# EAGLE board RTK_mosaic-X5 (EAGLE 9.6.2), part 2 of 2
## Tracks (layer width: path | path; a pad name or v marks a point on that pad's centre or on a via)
1.8V  (via drill 0.3)
  Top 0.254: C60.1 51.88,78.02 51.88,86.61 52.69,87.42 U13.1 | R18.2 92.9,89.11 | 92.9,89.11 93.88,89.11 94.41,89.65 U11.5 | U11.1 92.91,89.1 92.9,89.11
  Top 0.406: v63.18,74.42 57.25,74.42 C62.1 C60.1
  Top 0.61: U8.AC4 89.85,86.36 1V8.1 90.07,89.11 R18.2
  Route15 0.61: 1V8.1 84.77,87.63 71.56,74.42 v63.18,74.42
2V8
  Top 0.152: U8.M23 U8.N23 63.18,71.12 2V8.1
3.3V  (via drill 0.3)
  Top 0.152: U7.17 135.09,62.87 v135.06,62.84
  Top 0.254: R16.2 127.74,52.2 v127.44,52.2 | R59.1 v8.57,16.51 | R58.1 v132.78,70.23 | R57.1 v131.25,75.69 | U17.1 100.53,88.89 v100.52,88.9 | U17.5 102.03,88.91 v102.04,88.9 | U18.1 104.34,88.89 v104.33,88.9 | U4.P2 v111.19,88.9
  Top 0.406: C1.1 109.74,78.32 R3.2 | v122.24,28.07 122.24,27.09 C3.1 C4.1 122.28,24.42 v122.24,24.38 U2.16 | U2.4 v126.05,18.8 | U6.1 73.22,39.03 73.3,38.95
  Top 0.61: J4.2 76.38,13.2 v76.71,13.53 77.15,13.97 80.84,13.97 81.34,14.48 C56.1
  Top 0.813: 3V3.1 77.57,38.95 C15.1 C14.1 73.3,38.95 | v141.29,57.15 C32.1 | C32.1 C21.1 FB2.1 | R21.2 v131.89,57.15 131.09,57.15 R49.2 | 112.42,76.62 C1.1 111.44,67.31 110.35,66.22 U1.2 | 112.42,76.62 v112.46,76.58 | 112.42,76.62 C2.1 114.45,76.62 v114.49,76.58 | VCCIO.1 117.79,86.69 117.79,88.01 | 117.79,88.01 v117.79,88.9 v119.06,88.9 | v82.61,28.07 v82.61,26.67 82.61,16.04 82.23,15.66 C56.1 | C32.1 R29.2 | C41.1 117.75,88.05 117.79,88.01
  Route15 0.152: v135.06,62.84 135.06,57.15
  Route15 0.254: v8.57,16.51 10.35,18.29 26.86,18.29 40.83,4.32 53.53,4.32 62.74,13.53 v76.71,13.53 | v132.78,70.23 131.89,70.23 | v131.25,75.69 129.67,74.11
  Route15 0.813: v126.05,18.8 126.05,19.68 122.24,23.5 v122.24,24.38 v122.24,28.07 122.24,38.1 | 3V3.1 82.61,38.1 | 82.61,38.1 122.24,38.1 | 122.24,38.1 129.22,38.1 131.89,40.77 131.89,52.2 | v141.29,57.15 135.06,57.15 v131.89,57.15 | v112.46,76.58 v114.49,76.58 127.19,76.58 | 131.89,52.2 v131.89,57.15 | v127.44,52.2 131.89,52.2 | 125.41,88.9 127.19,87.12 127.19,76.58 | 125.41,88.9 v119.06,88.9 v117.79,88.9 v111.19,88.9 v104.33,88.9 v102.04,88.9 v100.52,88.9 | 125.41,88.9 125.41,97.79 126.68,99.06 132.78,99.06 | 132.78,99.06 140.67,99.06 J9.11 | J9.13 132.75,99.03 132.78,99.06 | 127.19,76.58 129.67,74.11 131.89,71.88 131.89,70.23 v131.89,57.15 | v82.61,26.67 v82.61,28.07 82.61,38.1
  Bottom 0.152: I2C.2 75.88,14.35 v76.71,13.53
  Bottom 0.813: ESP2.1 104.2,76.58 v112.46,76.58 v114.49,76.58
  cutout Route15: 22.8,91.06 arc-90 24.7,89.15 arc-90 22.8,87.25 arc-90 20.89,89.15 arc-90
3.3V_SW  (via drill 0.3)
  Top 0.152: U8.B8 84.14,57.78 72.07,57.78 | R56.1 34.23,87.03 v34.23,88.27 | R55.1 R15.2 | U14.1 45.92,88.15 47.42,89.65 U14.5
  Top 0.254: v45.91,77.09 45.81,76.99 U9.17 | U16.1 96.72,88.89 v96.71,88.9 | v44.01,87.25 44.89,87.25 45.07,87.42 U14.1 | U15.1 48.88,87.42 v48.7,87.25
  Top 0.406: J3.4 45.62,13.88 44.77,14.73 44.77,15.62 C18.1 44.75,15.68 D34.1 42.16,15.68 v42.1,15.62 42.1,17.02 41.76,17.36 R47.2 | U3.1 73.05,44.11 73.13,44.03 | U8.C18 v72.07,69.85 | C63.1 98.02,83.22 v97.35,82.55 97.35,76.33 RDY1.1 | R46.2 v52.13,18.41 55.18,18.41 55.44,18.16 R17.2
  Top 0.61: C54.1 68.77,53.34 69.53,54.1 U8.A20 U8.B20 U8.C20 | C53.1 70.42,53.34 70.8,53.72 U8.A19 U8.B19 U8.C19 | C46.1 U8.A18 U8.B18 72.07,57.78 U8.C18
  Top 0.813: C7.1 C6.1 73.13,44.03 | C7.1 77.57,44.03 3V3_SW.1 | C7.1 76.39,50.29 75.03,51.65 C46.1 C53.1 C54.1 | v49.34,15.62 48.11,15.62 C19.1 C20.1 C18.1 | FB1.1 48.83,70.32 v48.83,68.58 | v37.02,67.31 R20.2 | C5.1 v45.91,77.09 | C11.1 v45.91,78.74 | R15.2 v44.01,87.25 | C58.1 v42.35,87.25
  Route15 0.813: 3V3_SW.1 78.42,40.64 77.53,39.75 60.26,39.75 | v42.1,15.62 v49.34,15.62 v52.13,18.41 60.26,26.54 60.26,39.75 | 60.26,39.75 58.1,41.91 58.1,51.31 48.83,60.58 v48.83,68.58 45.91,68.58 | 45.91,68.58 38.29,68.58 v37.02,67.31 | 45.91,68.58 v45.91,77.09 v45.91,78.74 45.91,87.25 | 45.91,87.25 v44.01,87.25 v42.35,87.25 34.73,87.25 34.23,87.76 v34.23,88.27 34.23,89.28 32.07,91.44 26.37,91.44 J2.11 18.75,99.06 13.63,99.06 J2.13 | 45.91,87.25 v48.7,87.25
  Bottom 0.406: v72.07,69.85 74.61,69.85 87.31,82.55 v97.35,82.55 97.35,83.44 96.71,84.07 v96.71,88.9
5V  (via drill 0.3)
  Top 0.152: U6.5 67.84,40.98 67.09,40.23 67.09,39.05 | U3.5 67.97,46.06 67.09,45.19 67.09,44.13
  Top 0.406: U3.8 67.9,44.11 | U6.8 67.9,39.03 67.88,39.05
  Top 0.61: U8.A8 v84.77,53.34
  Top 0.813: 67.88,39.05 67.09,39.05 C17.1 62.33,38.95 60.64,40.64 5V.1 | 67.09,44.13 C9.1 | C9.1 C8.1 C10.1 61.06,44.03 5V.1 | F1.1 54.78,47.78 56.69,45.86 C57.+ 5V.1 | v56.83,73.41 v58.1,73.41 FB3.1 | v84.77,53.34 v83.63,53.34 82.87,53.34 82.23,52.7 C61.1 | v125.41,86.61 v124.14,86.61 122.86,86.61 VCCIO.3 | C9.1 67.07,44.11 67.9,44.11
  Route15 0.813: 5V.1 60.64,53.34 | 60.64,53.34 58.1,55.88 v58.1,73.41 v56.83,73.41 | 60.64,53.34 v83.63,53.34 v84.77,53.34 103.31,53.34 104.46,54.48 104.46,81.92 105.09,82.55 122.87,82.55 125.41,85.09 v125.41,86.61 v124.14,86.61
5V_RAW
  Top 0.813: U10.2 U10.1 29.72,54.17 30.3,54.75 C48.+ 32.93,54.98 C49.1 | C49.1 C50.1 | L1.1 37.78,53.38 C49.1
5V_RAW1
  Top 0.813: C16.+ 41.96,26.9 C51.1 C84.1 42.06,33.76 L4.1
  Top 1.905: U12.4 C16.+
!BOOT!  (via drill 0.3)
  Top 0.152: R16.1 R19.2 v134.3,51.18 | Q1.6 115.9,18.91 116.01,18.8 116.4,18.8 v116.52,18.92 | v121.6,20.32 v139.38,20.32
  Bottom 0.152: BOOT_SW.1 TP_BOOT.1 v139.38,20.32 139.38,46.1 v134.3,51.18 | v116.52,18.92 120.2,18.92 v121.6,20.32
!RESET!  (via drill 0.3)
  Top 0.152: MOSAIC_RST.4 v97.47,43.18 102.55,38.1 v102.55,21.59 | U1.3 106.29,64.95 v106.24,64.9 106.24,75.22 C31.1 R3.1 | Q1.3 114.6,21.86 114.36,22.1 113.22,22.1 v112.71,21.59
  Bottom 0.152: v97.47,43.18 100.01,45.72 100.01,64.01 100.9,64.9 v106.24,64.9 | RESET_SW.1 112.71,13.22 v112.71,21.59 v102.55,21.59 | MOSAIC_RST.4 MOSAIC_RST.2
ANT1
  Top 0.318: ANT1.SIG 69.53,94.69 D17.1 arc90 69.49,94.5 L3.2 69.49,83.86 arc90 U8.AC20
ANT2
  Top 0.318: U8.V23 64.92,77.47 arc-90 62.38,80.01 R53.2 62.37,81.3 D2.1 62.33,85.38 L2.1 62.42,87.08 ANT2.FEED
CH340-DTR  (via drill 0.3)
  Top 0.152: R4.2 117.72,21.24 v116.78,21.24 Q1.1 115.9,22.21 115.25,22.86 DTR.1 | U2.13 126.05,21.84 125.41,21.21 v120.33,21.21
  Bottom 0.152: v120.33,21.21 116.81,21.21
  Bottom 0.267: 116.81,21.21 v116.78,21.24
CH340-RTS  (via drill 0.3)
  Top 0.152: R5.2 111.51,19.4 v113.47,19.4 Q1.4 114.6,18.43 115.25,17.78 RTS.1 | U2.14 124.78,22.23 124.4,21.85 119.96,21.85 119.19,21.08 v119.19,19.43
  Bottom 0.152: 119.16,19.4 v113.47,19.4
  Bottom 0.267: v119.19,19.43 119.16,19.4
CH340-RXI  (via drill 0.3)
  Top 0.152: U2.3 124.78,15.88 TX.1 | v120.97,49.66 120.21,49.66 119.7,50.16 119.7,60.33 123.05,63.68 U1.35
  Bottom 0.152: v120.97,49.66 120.97,44.58 127.19,38.35 127.19,17.27 125.41,15.49 TX.1
CH340-TXO  (via drill 0.3)
  Top 0.152: U2.2 123.51,15.88 RX.1 | v120.33,50.8 120.33,60.33 122.42,62.41 U1.34
  Bottom 0.152: v120.33,50.8 120.33,44.45 126.68,38.1 126.68,18.03 123.89,15.24 RX.1
COM2_CTS
  Top 0.152: U8.J1 COM2_CTS.1
COM2_RTS
  Top 0.152: U8.G1 COM2_RTS.1
COM2_RX
  Top 0.152: U8.F1 COM2_RX.1
COM2_TX
  Top 0.152: U8.H1 COM2_TX.1
COM3_CTS
  Top 0.152: U8.N1 97.47,71.12 COM3_CTS.1
COM3_RTS
  Top 0.152: U8.L1 97.47,68.58 COM3_RTS.1
COM3_RX
  Top 0.152: U8.K1 COM3_RX.1
COM3_TX
  Top 0.152: U8.M1 96.96,69.85 98.23,71.12 COM3_TX.1
COM4_RX  (via drill 0.3)
  Top 0.152: U8.D3 91.76,59.05 96.58,59.05 100.52,55.12 v101.79,55.12 | v133.03,47.88 R52.2
  Bottom 0.152: v101.79,55.12 133.41,55.12 133.67,54.86 133.67,48.51 v133.03,47.88
COM4_TX  (via drill 0.3)
  Top 0.152: U8.E3 91.76,60.33 96.2,60.33 100.65,55.88 v101.79,55.88 | v132.91,55.63 132.1,55.63 130.96,54.48 R51.2
  Bottom 0.152: v101.79,55.88 131.64,55.88 131.89,55.63 v132.91,55.63
D+_ESP32  (via drill 0.3)
  Top 0.152: 127.7,8.89 J1.A6 127.7,5.33 127.95,5.08 128.46,5.08 128.7,5.32 J1.B6
  Top 0.267: 127.7,8.89 127,9.59 D10.1 127,11.37 v127.19,11.56 | v127.44,16.51 127.44,16.63 127.32,16.76 U2.5
  Bottom 0.267: v127.44,16.51 127.7,16.26 127.7,12.06 v127.19,11.56
D+_MOSAIC
  Top 0.267: J6.A6 104.84,5.2 104.97,5.08 105.6,5.08 105.84,5.32 J6.B6 105.84,7.8 107.25,9.21 107.25,11.05 106.04,12.26 D8.1 106.04,13.78 105.38,14.45 105.38,14.95 105.49,15.07 T1.A2
D+_MOSAIC_T
  Top 0.267: U8.A5 88.58,55.63 105.35,38.86 105.35,18.16 105.49,18.02 T1.A1
D-_ESP32  (via drill 0.3)
  Top 0.152: J1.B7 127.19,6 v127.19,7.11 | 128.2,8.89 128.2,7.24 v128.33,7.11 128.2,6.98 J1.A7
  Top 0.267: 128.2,8.89 128.9,9.59 D10.3 128.9,11.37 v128.71,11.56 | v128.46,16.51 128.59,16.64 U2.6
  Bottom 0.152: v128.33,7.11 v127.19,7.11
  Bottom 0.267: v128.46,16.51 128.21,16.26 128.21,12.06 v128.71,11.56
D-_MOSAIC
  Top 0.267: J6.A7 105.34,6.99 | 105.34,6.99 105.34,8 106.73,9.38 106.73,10.82 105.87,11.68 104.33,11.68 104.14,11.87 D8.3 104.14,13.78 104.81,14.45 104.81,14.95 104.69,15.07 T1.B2 | J6.B7 104.34,6.74 104.58,6.99 105.34,6.99
D-_MOSAIC_T
  Top 0.267: T1.B1 104.69,17.95 104.84,18.1 104.84,38.61 87.57,55.88 U8.A6
ESP2_TX
  Top 0.152: U1.24 125.7,49.53 R48.1 R52.1
ESP4_RX
  Top 0.152: U1.26 126.48,52.25 127.06,52.83 127.06,54.23 127.32,54.48 R51.1
ESP5_ERST  (via drill 0.3)
  Top 0.152: U1.29 128.3,56.06 R49.1 128.37,57.19 129.6,58.42 v130.49,58.42 | U7.32 139.74,67.79 139.89,67.94 v140.65,67.94
  Bottom 0.152: v130.49,58.42 133.03,60.96 139.38,60.96 141.16,62.74 141.16,67.44 v140.65,67.94
ESP12_LED_WIFI  (via drill 0.3)
  Top 0.152: v104.58,49.4 104.58,50.71 R50.1 104.85,50.98 U1.14 | v10.22,15.98 R28.1
  Bottom 0.152: v104.58,49.4 104.58,47.62 97.6,40.64 85.79,40.64 58.48,13.34 16.68,13.34 14.03,15.98 v10.22,15.98
ESP14_SCL  (via drill 0.3)
  Top 0.152: R_SCL.1 71.35,16.38 v70.8,16.38 | J4.4 73.2,11.93 72.71,11.43 SCL2.1 | v106.11,52.32 107.45,52.32 U1.13 | v73.98,16.38 73.98,26.04 89.85,41.91 v96.96,41.91 | v100.77,45.72 100.77,51.56 101.54,52.32 v103.95,52.32 104.3,52.68 104.3,77.64 106.95,80.29 107.52,80.29 111.69,84.47 U4.P3
  Bottom 0.152: v73.98,16.38 v70.8,16.38 SCL2.1 | v103.95,52.32 v106.11,52.32 | v100.77,45.72 v96.96,41.91
ESP14_SCL_IO  (via drill 0.3)
  Top 0.152: R_SCL_IO.1 110.3,85.98 v110.68,85.6 | U4.P6 111.69,92.27 D26.1
  Top 0.406: J13.4 112.88,94.53 111.75,93.4 D26.1
  Bottom 0.152: v110.68,85.6 112.88,87.8 J13.4
ESP15_LED_BT  (via drill 0.3)
  Top 0.152: v105.22,48.51 107.45,48.51 U1.16 | R36.1 13.23,14.82 v13.65,15.24
  Bottom 0.152: v13.65,15.24 15.94,12.95 58.61,12.95 85.92,40.26 97.98,40.26 105.22,47.5 v105.22,48.51
ESP15_SDA  (via drill 0.3)
  Top 0.152: 78.42,15.66 78,15.66 74.36,19.3 74.36,26.02 89.74,41.4 v97.6,41.4 | 78.42,15.66 R_SDA.1 | J4.3 75.38,11.04 75.59,10.83 80.36,10.83 SDA2.1 | v78.42,15.7 78.42,15.66 | v124.14,48.39 125.47,48.39 U1.23 | v101.28,45.09 101.28,51.56 101.54,51.82 104.33,51.82 105.09,52.58 v105.09,52.96 104.58,53.47 104.58,77.52 107.07,80.01 107.63,80.01 112.19,84.57 U4.P4
  Bottom 0.152: SDA2.1 78.42,13.97 v78.42,15.7 | v105.09,52.96 119.57,52.96 v124.14,48.39 | v101.28,45.09 v97.6,41.4
ESP15_SDA_IO  (via drill 0.3)
  Top 0.152: R_SDA_IO.1 110.3,84.33 v110.68,84.71 | U4.P5 112.19,91.05 112.59,91.44 113.47,91.44 114.36,92.33 D25.1
  Top 0.406: D25.1 115.18,93.27 116.38,94.47 J13.3
  Bottom 0.152: v110.68,84.71 116.38,90.41 J13.3
ESP18_MDIO  (via drill 0.3)
  Top 0.152: U7.11 133.3,66.79 v133.29,66.8 | v130.87,63.5 131.34,63.5 131.89,62.95 R21.1 131.09,60.54 127.88,57.33 U1.30
  Bottom 0.152: v133.29,66.8 130.87,64.39 v130.87,63.5
ESP19_TXD0  (via drill 0.3)
  Top 0.152: U1.31 126.61,58.6 126.81,58.8 126.81,60.07 128.71,61.98 v130.24,61.98 | U7.24 138.59,62.58 v138.37,62.36
  Bottom 0.152: v130.24,61.98 130.37,61.85 137.86,61.85 v138.37,62.36
ESP21_TXEN  (via drill 0.3)
  Top 0.152: U1.33 127.24,61.14 128.59,62.48 v130.87,62.48 | v137.73,62.74 138.09,63.1 U7.23
  Bottom 0.152: v137.73,62.74 137.22,62.23 131.13,62.23 v130.87,62.48
ESP22_TXD1  (via drill 0.3)
  Top 0.152: U1.36 126.63,64.95 128.59,62.99 v130.24,62.99 | v140.53,64.26 139.25,64.26 U7.25
  Bottom 0.152: v130.24,62.99 131.51,62.99 131.89,63.37 139.64,63.37 v140.53,64.26
ESP23_MDC
  Top 0.152: U1.37 126.5,66.22 128.59,64.14 131.89,64.14 132.52,64.77 132.52,65.41 133.41,66.29 U7.12
ESP25_RXD0  (via drill 0.3)
  Top 0.152: U1.10 108.96,56.06 v109.28,56.39 | v135.19,56.26 R30.1
  Bottom 0.152: v109.28,56.39 109.41,56.26 133.03,56.26 133.54,55.75 134.68,55.75 v135.19,56.26
ESP26_RXD1  (via drill 0.3)
  Top 0.152: U1.11 108.57,54.79 v110.81,57.02 | R31.1 133.54,56.72 v133.92,56.34
  Bottom 0.152: v110.81,57.02 111.16,56.67 133.03,56.67 133.36,56.34 v133.92,56.34
ESP27_CRSDV  (via drill 0.3)
  Top 0.152: U1.12 109.08,53.52 v110.17,54.61 | v132.91,54.61 133.92,55.63 135.57,55.63 136.08,56.13 136.08,57.06 136.84,57.82 R32.1
  Bottom 0.152: v110.17,54.61 v132.91,54.61
ESP32_RF
  Top 0.318: ESP32_RF.SIG 82.23,94.67 D3.1 82.18,92.44 J8.FEED
ESP32_TX  (via drill 0.3)
  Top 0.152: v102.55,59.31 103.34,60.1 103.34,81.76 101.03,84.07 U17.2 | v106.11,58.67 107.45,58.67 U1.8
  Bottom 0.152: v106.11,58.67 105.35,57.91 103.31,57.91 102.55,58.67 v102.55,59.31
ESP32_TX_O
  Top 0.152: U17.7 101.03,91.32 101.16,91.44 102.17,91.44 102.37,91.64 D24.1
  Top 0.406: D24.1 102.37,95.61 J13.7
ESP33_RTS  (via drill 0.3)
  Top 0.152: v102.55,57.4 102.55,58.55 103.62,59.61 103.62,81.99 101.53,84.08 U17.3 | v106.11,57.4 107.45,57.4 U1.9
  Bottom 0.152: v102.55,57.4 v106.11,57.4
ESP33_RTS_O
  Top 0.152: U17.6 101.53,90.93 101.66,91.06 103.5,91.06 D23.1
  Top 0.406: D23.1 104.77,93.27 105.88,94.39 J13.6
ESP34_RX  (via drill 0.3)
  Top 0.152: v102.55,61.85 103.06,62.36 103.06,81.28 v102.43,81.92 | v106.11,61.09 107.47,61.09 U1.6 | U18.2 v104.84,84.33
  Bottom 0.152: v102.55,61.85 105.35,61.85 v106.11,61.09 | v102.43,81.92 v104.84,84.33
ESP34_RX_I  (via drill 0.3)
  Top 0.152: U18.7 104.84,91.11 v104.87,91.14
  Top 0.406: D28.1 98.81,95.56 J13.8
  Bottom 0.152: v104.87,91.14 99.93,91.14 98.88,92.19 J13.8
ESP35_CTS  (via drill 0.3)
  Top 0.152: v103.44,58.67 103.95,59.18 103.95,82.68 105.34,84.07 U18.3 | v106.11,59.94 107.45,59.94 U1.7
  Bottom 0.152: v103.44,58.67 104.84,58.67 v106.11,59.94
ESP35_CTS_I
  Top 0.152: U18.6 105.34,90.8 105.73,91.19 106.36,91.19 107.51,92.33 D27.1
  Top 0.406: D27.1 108.32,93.4 109.38,94.46 J13.5
ESP36  (via drill 0.3)
  Top 0.152: v105.47,63.63 105.53,63.68 U1.4
  Bottom 0.152: ESP36.1 101.28,61.98 101.79,62.48 104.33,62.48 v105.47,63.63
ESP39  (via drill 0.3)
  Top 0.152: U1.5 105.91,62.41 105.35,61.85 v105.35,60.45
  Bottom 0.152: v105.35,60.45 102.68,60.45 102.04,59.82 101.54,59.82 101.28,59.56 ESP39.1
ESP_REFCLK  (via drill 0.3)
  Top 0.152: R19.1 128.17,50.98 U1.25 123.96,50.98 122.87,52.07 v122.87,59.69 | v133.41,67.77 134.45,67.77 U7.9
  Bottom 0.152: v122.87,59.69 127.95,59.69 129.6,61.34 129.6,63.96 v133.41,67.77
ETHER_!RST!  (via drill 0.3)
  Top 0.152: U9.32 39.84,81.66 v39.56,81.94 | v42.35,82.93 R22.2 | U8.F2 91.76,62.87 90.61,62.87 90.11,63.37 v88.58,63.37 | v53.02,63.37 53.02,68.2 49.53,71.69 v49.15,71.69
  Bottom 0.152: v39.56,81.94 41.34,81.94 42.33,82.93 v42.35,82.93 44.89,82.93 49.15,78.68 v49.15,71.69 | v88.58,63.37 v53.02,63.37
ETHER_CLK  (via drill 0.3)
  Top 0.152: U8.AA2 91.76,80.64 90.49,80.64 90.11,80.26 90.11,78.99 81.85,70.74 v81.85,67.56 | U9.9 39.84,74.65 40.2,74.3 43.24,74.3 44.64,75.69 50.61,75.69 56.45,69.85 v56.96,69.85
  Bottom 0.152: v81.85,67.56 81.47,67.18 57.59,67.18 57.34,67.44 57.34,69.47 v56.96,69.85
ETHER_CRSDV  (via drill 0.3)
  Top 0.152: v55.05,66.67 54.93,66.8 54.93,68.83 49.85,73.91 45.4,73.91 44.01,72.52 v44.01,72.26 | U8.N2 91.76,71.75 89.47,71.75 85.28,67.56 v85.28,65.66 | U9.18 44.66,77.49 v44.77,77.6
  Bottom 0.152: v85.28,65.66 85.28,65.53 85.03,65.28 55.69,65.28 55.44,65.53 55.44,66.29 v55.05,66.67 | v44.01,72.26 44.01,76.83 v44.77,77.6
ETHER_MDC  (via drill 0.3)
  Top 0.152: v83.38,66.8 83.38,70.36 89.85,76.83 91.76,76.83 U8.V2 | v41.59,73.28 43.24,73.28 45.02,75.06 50.24,75.06 56.07,69.23 56.07,68.71 v56.2,68.58 | U9.12 41.34,75.18 v41.59,74.93
  Bottom 0.152: v83.38,66.8 82.99,66.42 56.83,66.42 56.58,66.67 56.58,68.2 v56.2,68.58 | v41.59,74.93 | v41.59,73.28 v41.59,74.93
ETHER_MDIO  (via drill 0.3)
  Top 0.152: U8.W2 91.76,78.11 90.11,78.11 82.61,70.61 v82.61,67.18 | v56.58,69.24 50.48,75.34 44.77,75.34 43.24,73.81 v40.96,73.81 40.93,73.79 39.18,73.79 37.02,71.63 R20.1 | v40.83,75.56 40.83,76.35 U9.11
  Bottom 0.152: v56.58,69.24 56.96,68.86 56.96,67.08 57.21,66.83 82.33,66.83 82.61,67.11 v82.61,67.18 | v40.96,73.81 40.96,75.44 v40.83,75.56
ETHER_RXD0  (via drill 0.3)
  Top 0.152: U8.R2 91.76,73.03 89.85,73.03 84.65,67.82 v84.65,66.04 | v55.44,67.31 55.31,67.44 55.31,68.96 49.97,74.3 45.28,74.3 43.24,72.26 v42.74,72.26 | v43.5,75.44 43.34,75.59 U9.16
  Bottom 0.152: v84.65,66.04 84.26,65.66 62.29,65.66 56.07,65.66 55.82,65.91 55.82,66.93 v55.44,67.31 | v43.5,75.44 43.5,73.03 v42.74,72.26
ETHER_RXD1  (via drill 0.3)
  Top 0.152: U8.T2 91.76,74.3 90.23,74.3 84.01,68.07 v84.01,66.42 | v42.23,72.77 43.24,72.77 45.15,74.68 50.1,74.68 55.69,69.09 55.69,68.07 v55.82,67.94 | v42.86,74.93 42.84,74.95 U9.15
  Bottom 0.152: v84.01,66.42 84.01,66.35 83.73,66.07 56.42,66.07 56.2,66.29 56.2,67.56 v55.82,67.94 | v42.86,74.93 42.23,74.3 v42.23,72.77
ETHER_RXER  (via drill 0.3)
  Top 0.152: U8.M2 91.76,70.48 89.09,70.48 86.04,67.44 v86.04,65.28 | v44.89,72.26 44.89,72.9 45.53,73.53 49.72,73.53 54.55,68.71 54.55,66.17 v54.67,66.04 | U9.20 v44.76,78.49 v44.77,78.49
  Bottom 0.152: v86.04,65.28 85.66,64.9 55.31,64.9 55.05,65.15 55.05,65.66 v54.67,66.04 | v44.77,78.49 45.28,77.98 45.28,72.64 v44.89,72.26
ETHER_TXD0  (via drill 0.3)
  Top 0.152: U9.24 44.87,80.49 v44.89,80.52 | v87.31,64.39 89.6,66.67 91.76,66.67 U8.J2 | v47.43,72.14 47.94,72.64 49.59,72.64 53.78,68.45 53.78,64.9 v54.04,64.64
  Bottom 0.152: v44.89,80.52 45.78,80.52 47.43,78.87 v47.43,72.14 | v87.31,64.39 87.06,64.14 54.42,64.14 54.04,64.52 v54.04,64.64
ETHER_TXD1  (via drill 0.3)
  Top 0.152: U8.H2 91.76,65.41 89.39,65.41 v87.95,63.96 | v53.53,64.01 53.4,64.14 53.4,68.33 49.53,72.2 48.39,72.2 v48.32,72.14 | v43.5,82.17 43.34,82.01 U9.25
  Bottom 0.152: v87.95,63.96 87.95,63.93 87.77,63.75 53.78,63.75 v53.53,64.01 | v48.32,72.14 48.32,78.74 44.89,82.17 v43.5,82.17
ETHER_TXEN  (via drill 0.3)
  Top 0.152: U8.L2 91.76,69.22 88.71,69.22 86.68,67.18 v86.68,64.77 | v44.89,79.63 44.53,79.99 U9.23 | v46.93,72.77 47.18,73.03 49.72,73.03 54.19,68.55 54.19,65.59 54.29,65.49 v54.29,65.41
  Bottom 0.152: v86.68,64.77 86.42,64.52 55.05,64.52 54.29,65.28 v54.29,65.41 | v46.93,72.77 46.93,78.87 46.16,79.63 v44.89,79.63
GND  (via drill 0.3)
  Top 0.152: U9.1 39.84,80.49 U9.GND
  Top 0.254: U7.GND 138.59,67.79 U7.1 138.59,68.85 138.83,69.09 v139.38,69.09 | U9.1 38.83,80.49 v38.29,81.03
  Bottom 0.152: SHLD1.1 127.94,3.68 v126.56,3.68 | SHLD2.1 104.98,3.81 v103.82,3.81
  other vias: 28.89,73.66 28.89,72.39 28.89,71.12 28.89,69.85 26.35,68.58 26.35,67.31 26.35,66.04 26.35,64.77 26.35,63.5 26.35,62.23 26.35,60.96 26.35,59.69 27.62,59.69 27.62,60.96 27.62,62.23 27.62,63.5 27.62,64.77 27.62,66.04 27.62,67.31 27.62,68.58 28.89,68.58 28.89,67.31 28.89,66.04 28.89,64.77 28.89,63.5 28.89,62.23 28.89,60.96 28.89,59.69 28.26,60.33 26.99,60.33 26.99,61.59 28.26,61.59 28.26,62.87 26.99,62.87 26.99,64.14 26.99,65.41 26.99,66.67 28.26,67.94 26.99,67.94 28.26,66.67 28.26,65.41 28.26,64.14 26.99,59.05 28.26,59.05 27.62,58.42 26.35,58.42 28.89,58.42 41.59,59.69 42.86,59.69 44.13,59.69 45.4,59.69 46.67,59.69 45.4,58.42 46.67,58.42 44.13,58.42 42.23,59.05 43.5,59.05 44.77,59.05 44.77,57.78 46.04,59.05 46.04,57.78 40.32,59.69 39.05,59.69 39.05,58.42 40.32,58.42 40.96,59.05 39.69,59.05 39.69,57.78 40.96,57.78 74.61,36.07 76.52,36.07 76.39,41.02 74.49,41.02 72.96,46.1 65.09,41.15 63.18,41.15 66.99,36.07 66.99,41.15 32.7,61.59 31.81,61.59 33.59,61.59 37.78,57.78 41.08,54.48 49.21,44.45 49.21,45.47 49.21,43.43 73.6,99.19 73.6,100.46 73.6,97.92 73.34,96.65 72.07,96.65 70.8,95.38 70.8,93.6 70.8,91.82 70.8,90.17 68.26,91.82 68.26,93.34 67.12,95.38 68.26,85.09 66.99,96.65 65.72,96.77 65.47,99.19 65.47,97.92 65.47,100.46 78.17,99.06 86.3,99.06 78.17,100.46 78.17,97.54 86.3,97.41 86.3,100.46 79.69,96.52 79.82,94.61 84.77,96.65 83.88,95.5 83.38,94.61 83.5,92.46 84.77,90.81 83.63,89.03 80.96,89.03 82.23,89.03 79.82,90.68 80.96,92.46 46.55,18.54 44.77,18.54 48.2,18.54 43.5,13.97 43.5,11.18 40.83,37.72 45.02,33.53 78.42,12.45 78.42,11.43 81.34,18.54 124.14,13.46 131.76,13.46 127.95,11.56 30.16,77.47 35.24,88.52 34.48,90.81 121.35,17.53 126.05,68.45 125.03,68.45 107,68.45 108.01,68.45 115,62.1 112.71,59.69 112.71,62.1 117.41,59.69 117.41,62.1 115,57.28 117.41,57.28 112.71,57.28 108.78,49.66 107.63,79.5 111.44,79.5 113.47,79.5 102.55,13.72 108.9,13.46 131.25,6.99 108.39,6.99 100.77,7.24 125.29,27.05 125.29,25.4 33.08,73.66 68.26,88.9 61.02,86.49 70.8,87.63 70.8,86.36 70.8,85.09 67.63,83.19 67.63,81.92 68.9,81.92 70.17,81.92 71.44,81.92 71.44,83.19 37.91,85.98 33.08,81.92 123.63,7.24 105.09,13.97 56.2,88.27 55.05,86.36 53.66,79.38 49.97,78.74 49.97,76.2 31.56,82.93 101.79,50.8 82.23,48.77 130.87,78.74 143.19,78.74 144.46,75.69 136.21,75.69 128.46,68.58 145.73,69.72 141.67,64.77 141.29,61.72 72.96,41.02 70.8,42.93 69.53,42.93 70.17,42.93 72.07,42.93 72.07,42.16 71.44,42.93 71.44,42.16 70.8,42.16 70.17,42.16 69.53,42.16 70.8,47.24 70.17,47.24 69.53,47.24 72.07,47.24 72.07,48.01 70.8,48.01 71.44,48.01 71.44,47.24 69.53,48.01 70.17,48.01 70.8,37.08 70.17,37.08 69.53,37.08 72.07,37.08 71.44,37.08 70.8,37.85 69.53,37.85 70.17,37.85 71.44,37.85 72.07,37.85 66.36,83.19 66.36,80.64 66.36,76.83 67.63,80.64 67.63,62.87 66.36,56.52 67.63,56.52 66.36,62.87 63.18,62.23 93.03,80.64 86.68,83.19 76.52,81.92 91.76,83.19 91.76,79.38 91.76,75.56 93.03,76.83 93.03,66.67 93.03,71.75 93.03,62.87 91.76,57.78 87.95,56.52 86.68,57.78 85.41,56.52 73.98,56.52 75.25,56.52 91.76,61.59 80.96,73.66 83.5,76.2 86.3,78.99 54.29,62.23 56.83,62.23 60.64,62.23 70.8,62.23 73.34,62.23 75.88,62.23 78.42,62.23 80.96,62.23 83.5,62.23 70.8,77.47 73.34,77.47 75.88,77.47 88.58,62.23 113.86,86.87 124.52,90.68 40.32,67.44 41.97,67.44 43.62,67.44 45.28,67.44 48.83,26.67 48.83,27.56 48.83,25.78 134.56,71.5 141.67,66.42 128.46,66.93 128.46,65.28 142.94,61.72 103.82,16.51 103.82,20.32 103.82,24.13 106.36,16.51 106.36,20.32 106.36,24.13 103.82,27.94 106.36,27.94 106.36,31.75 103.82,31.75 106.36,35.56 102.55,43.18 103.82,35.56 101.28,40.64 105.09,40.64 97.47,44.45 98.74,46.99 94.93,46.99 91.12,50.8 91.12,54.61 133.03,49.53 41.59,78.74 136.84,66.04 39.05,72.39 127.95,58.42 79.69,76.2 82.23,78.74 78.42,80.01 77.15,78.74 67.63,76.83 67.63,78.11 66.36,78.11 66.36,79.38 67.63,79.38 61.28,83.95 65.98,89.92 68.26,90.17 70.8,88.9 60.13,85.34 65.72,85.09 61.28,82.55 61.4,80.01 61.79,78.61 62.93,77.22 64.45,76.58 64.33,78.49 63.31,79.76 63.69,81.28 63.56,83.31 63.82,85.09 61.02,88.65 61.02,92.2 62.29,92.2 63.69,92.2 64.96,90.55 63.94,88.65 58.99,81.28 81.98,54.61 58.99,88.65 58.99,90.42 58.99,91.95 64.96,92.2 58.99,83.82 58.99,86.36 58.99,78.74 61.4,77.09 61.4,75.44 86.04,62.23 84.77,69.85 87.31,72.39 89.85,74.93 80.96,69.85 77.66,69.6 73.34,67.82 70.42,67.82 67.63,67.94 66.36,67.94 59.37,69.85 67.63,70.48 67.63,73.03 77.15,73.66 69.53,73.03 71.82,73.28 66.36,75.56 67.63,75.56 63.94,75.44 70.29,75.44 74.61,71.12 73.34,74.93 55.56,73.66 96.2,49.53 122.87,60.96 121.6,58.42 122.87,50.8 121.6,53.34 130.49,60.96 127.32,62.87 133.03,68.58 123.63,58.42 123.63,53.34 51.24,86.36 47.43,86.36 55.18,79.38 56.32,82.3 43.5,90.17 115.51,90.93 105.85,86.61 102.04,86.61 94.17,86.74 110.68,86.49 98.23,88.9 75.88,67.82 79.44,71.5 55.05,89.28 51.24,89.28 52.51,74.55 54.29,72.77 56.2,70.87 59.37,67.69 63.18,67.69 39.05,74.93 44.77,76.2 99.76,83.19 41.08,88.14 40.07,92.46 43.62,92.33 50.36,92.46 53.91,92.46 89.6,92.33 93.66,93.6 97.22,93.6 100.65,93.6 104.08,93.6 107.51,93.6 111.06,93.6 114.49,93.6 118.05,93.6 43.12,17.91 39.43,17.91 53.78,17.78 50.36,17.91
  pour Top (isolate 0.203, rank 2): 4.76,0 4.76,50.42 17.59,50.42 18.73,51.56 18.73,78.85 14.88,82.7 14.88,84.3 13.65,85.47 13.65,93.09 11.62,95.12 4.76,95.12 4.76,101.6 147,101.6 147,0
  pour Bottom (isolate 0.203, rank 2): 4.76,0 4.76,50.42 17.59,50.42 18.73,51.56 18.73,78.85 14.88,82.7 14.88,84.3 13.65,85.47 13.65,93.09 11.62,95.12 4.76,95.12 4.76,101.6 147,101.6 147,0
  pour Route2 (isolate 0.203, rank 2): 4.76,0 4.76,50.42 17.59,50.42 18.73,51.56 18.73,78.85 14.88,82.7 14.88,84.3 13.65,85.47 13.65,93.09 11.62,95.12 4.76,95.12 4.76,101.6 147,101.6 147,0
  pour Route15 (isolate 0.203, rank 2): 4.76,0 4.76,50.42 17.59,50.42 18.1,50.93 18.73,51.56 18.73,52.45 18.73,78.87 17.34,80.26 14.92,82.68 14.92,83.82 14.92,84.2 14.41,84.71 13.65,85.47 13.65,90.04 13.65,93.09 12.26,94.49 11.62,95.12 8.45,95.12 4.76,95.12 4.76,101.6 147,101.6 147,0
  cutout Top: 22.8,91.06 arc-90 24.7,89.15 arc-90 22.8,87.25 arc-90 20.89,89.15 arc-90
  cutout Bottom: 22.8,91.06 arc-90 24.7,89.15 arc-90 22.8,87.25 arc-90 20.89,89.15 arc-90
  cutout Route2: 22.8,91.06 arc-90 24.7,89.15 arc-90 22.8,87.25 arc-90 20.89,89.15 arc-90
  pour Top (isolate 0.127): 77.41,88.27 77.41,101.6 87.06,101.6 87.06,88.27
  pour Top (isolate 0.127): 60.01,75.95 60.01,101.6 74.61,101.6 74.61,75.95
  cutout Top: 127.44,88.52 127.44,89.79 128.33,90.68 145.48,90.68 146.37,89.79 146.37,88.52 145.35,87.5 135.57,87.5 134.94,86.87 134.94,85.09 136.21,83.82 136.21,77.72 135.95,77.47 134.3,77.47 133.79,77.98 133.79,83.69 132.4,85.09 132.4,87 131.89,87.5 128.46,87.5
GND-ISO  (2 unrouted)
  Top 0.813: J9.S2 133.67,89.15 | 133.67,89.15 J9.S1 | 133.67,89.15 J9.8 133.67,84.84 134.94,83.57 J9.7 134.94,78.89 C42.1
  pour Top (isolate 0.406, rank 2): 4.76,93.85 11.11,93.85 12.38,92.58 12.38,84.96 13.68,83.7 13.68,82.2 17.46,78.42 17.46,52.32 16.7,51.56 4.76,51.56
  pour Route2 (isolate 0.203): 4.76,93.85 11.11,93.85 12.38,92.58 12.38,84.96 13.68,83.7 13.68,82.2 17.46,78.42 17.46,52.32 16.7,51.56 4.76,51.56
  pour Route15 (isolate 0.203): 4.76,93.85 11.11,93.85 12.38,92.58 12.38,84.96 13.68,83.7 13.68,82.2 17.46,78.42 17.46,52.32 16.7,51.56 4.76,51.56
  pour Bottom (isolate 0.406, rank 2): 4.76,93.85 11.11,93.85 12.38,92.58 12.38,84.96 13.68,83.7 13.68,82.2 17.46,78.42 17.46,52.32 16.7,51.56 4.76,51.56
GPIO_1  (via drill 0.3)
  Top 0.152: U8.AA4 v88.58,80.01
  Bottom 0.152: v88.58,80.01 U8.AA4 GPIO_1.1
GPIO_2
  Top 0.152: U8.L3 91.76,67.94 97.6,67.94 98.23,68.58 GPIO_2.1
LED_PVT  (via drill 0.3)
  Top 0.152: U8.A14 v77.15,54.61 | v22.16,17.53 R38.1
  Bottom 0.152: v77.15,54.61 77.15,49.53 80.96,45.72 80.96,38.86 59.37,17.27 24.59,17.27 24.39,17.47 22.22,17.47 v22.16,17.53
LED_RTK  (via drill 0.3)
  Top 0.152: U8.M3 v89.85,69.85 | v20.51,16.51 R39.1
  Bottom 0.152: v89.85,69.85 94.93,69.85 95.82,68.96 95.82,52.7 59.63,16.51 v20.51,16.51
LINK_ESP32  (via drill 0.3)
  Top 0.152: v140.65,66.8 139.23,66.8 U7.30
  Top 0.254: R25.2 129.6,71.5 | 129.6,71.5 v132.86,71.5 | R58.2 129.6,70.27 129.6,71.5
  Bottom 0.152: v132.86,71.5 137.56,66.8 v140.65,66.8
LINK_MOSAIC
  Top 0.152: U9.30 40.84,82.81 40.44,83.21 37.9,83.21 37.15,83.96 37.15,84.2 36.13,85.22 R6.2 R56.2
LOG_LED  (via drill 0.3)
  Top 0.152: U8.B2 93.66,55.88 v93.66,52.07 | v23.81,16.99 R37.1
  Bottom 0.152: v93.66,52.07 93.66,51.05 59.52,16.92 23.89,16.92 v23.81,16.99
MEAS
  Top 0.813: MEAS.4 46.55,50.68 D9.C D6.C D5.C D4.C
  Bottom 0.152: MEAS.4 MEAS.2
MOSAIC_!RST!
  Top 0.152: MOSAIC_RST.3 84.01,45.72 80.96,48.77 U8.A11
  Bottom 0.152: MOSAIC_RST.3 MOSAIC_RST.1
MOSAIC_CTS  (via drill 0.3)
  Top 0.152: v94.93,60.96 U8.E1 | U15.3 50.71,87.4 v50.71,83.82
  Bottom 0.152: v94.93,60.96 52.9,60.96 51.6,62.26 51.6,82.93 v50.71,83.82
MOSAIC_CTS_I
  Top 0.152: U15.6 50.73,92.07 50.99,92.33 D19.1
  Top 0.406: D19.1 51.81,93.4 52.88,94.47 J5.3
MOSAIC_EVENTA_1V8  (via drill 0.3)
  Top 0.152: v87.31,85.09 U8.AC6 | v52.51,86.36 53.66,86.36 54.04,86.75 U13.2
  Bottom 0.152: v87.31,85.09 87.31,85.05 73.41,71.14 56.79,71.14 52.51,75.42 v52.51,86.36
MOSAIC_EVENTA_I  (via drill 0.3)
  Top 0.152: R43.2 53.4,84.84 v53.91,85.34 | v53.91,89.28 54.04,89.41 U13.7 54.04,91.14 D15.1
  Top 0.406: D15.1 55.24,93.27 56.38,94.42 J5.2
  Bottom 0.152: v53.91,85.34 v53.91,89.28
MOSAIC_EVENTB_1V8  (via drill 0.3)
  Top 0.152: v86.04,85.09 U8.AC7 | U13.3 54.54,86.74 53.69,85.88 v53.02,85.88
  Bottom 0.152: v86.04,85.09 86.04,84.28 73.18,71.42 56.94,71.42 53.02,75.35 v53.02,85.88
MOSAIC_EVENTB_I  (via drill 0.3)
  Top 0.152: v55.18,85.22 R44.2 | U13.6 v54.54,88.52 v54.55,88.52
  Top 0.406: D13.1 59.88,94.31 J5.1
  Bottom 0.152: v55.18,85.22 55.56,85.6 55.56,88.52 | J5.1 59.88,94.49 55.56,90.17 55.56,88.52 | v54.55,88.52 55.56,88.52
MOSAIC_LOG_BTN  (via drill 0.3)
  Top 0.152: v89.85,67.31 U8.K3 | v97.47,88.39 97.22,88.14 U16.2
  Bottom 0.152: v97.47,88.39 97.83,88.04 97.83,82.1 97.42,81.69 87.21,81.69 84.77,79.25 84.77,72.39 v89.85,67.31
MOSAIC_LOG_BTN_I  (via drill 0.3)
  Top 0.152: R27.2 31.01,14.82 30.16,13.97 v30.16,12.47 | v86.04,39.37 86.04,40.64 v87.31,41.91 | U16.7 97.22,91.06 | J13.9 95.38,95.25 95.38,94.55 96.59,93.34 96.59,91.69 97.22,91.06 | v96.58,79.63 96.58,84.54 R23.2 99.12,87.08 99.12,90.55 98.62,91.06 97.22,91.06
  Top 0.406: D18.1 95.39,95.25 95.38,95.25
  Bottom 0.152: v30.16,12.47 30.26,12.57 44.13,12.57 58.74,12.57 85.53,39.37 v86.04,39.37 | v87.31,41.91 87.31,42.16 97.09,51.94 97.09,79.12 v96.58,79.63
MOSAIC_PPSO
  Top 0.152: U11.7 93.41,92.96 91.88,94.49 J13.10
  Top 0.406: D16.1 91.83,95.57 J13.10
MOSAIC_PPSO_1V8  (via drill 0.3)
  Top 0.152: v84.77,85.09 U8.AC8 | U11.2 93.41,88.53 v93.44,88.56
  Bottom 0.152: v84.77,85.09 86.04,86.36 91.25,86.36 v93.44,88.56
MOSAIC_RTS  (via drill 0.3)
  Top 0.152: v94.93,58.42 U8.C1 | v48.73,84.98 48.11,85.6 47.18,85.6 46.92,85.86 U14.3
  Bottom 0.152: v94.93,58.42 95.44,58.93 95.44,59.94 95.06,60.33 94.81,60.33 94.45,60.68 52.65,60.68 51.32,62.01 51.32,82.39 v48.73,84.98
MOSAIC_RTS_O
  Top 0.152: U14.6 46.92,91.94 47.31,92.33 D21.1
  Top 0.406: D21.1 48.12,93.27 49.38,94.53 J5.4
MOSAIC_RX  (via drill 0.3)
  Top 0.152: v94.93,57.15 U8.B1 | U15.2 v50.23,82.04
  Bottom 0.152: v94.93,57.15 94.93,57.33 92.14,60.12 52.17,60.12 50.74,61.55 50.74,81.53 v50.23,82.04
MOSAIC_RX_I  (via drill 0.3)
  Top 0.152: U15.7 50.23,89.49 49.65,88.9 v48.58,88.9
  Top 0.406: D20.1 42.3,95.54 J5.6
  Bottom 0.152: v48.58,88.9 47.94,88.9 42.38,94.46 J5.6
MOSAIC_TX  (via drill 0.3)
  Top 0.152: v94.91,59.67 94.89,59.69 U8.D1 | v47.94,85.09 46.93,85.09 46.42,85.59 U14.2
  Bottom 0.152: v94.91,59.67 94.18,60.4 52.41,60.4 51.04,61.77 51.04,81.99 v47.94,85.09
MOSAIC_TX_O
  Top 0.152: D22.1 46.42,91.76 U14.7
  Top 0.406: D22.1 45.86,95.6 J5.5
N$1
  Top 0.152: J1.B5 129.7,8.52 R1.2
N$2
  Top 0.152: J1.A5 126.7,8.02 R2.2
N$3
  Bottom 0.152: J9.14 130.98,97.03 131.64,97.03 132.03,97.42 LINK.1
N$4
  Top 0.152: Q1.2 115.25,22.23 115,22.48 111.7,22.48 111.44,22.23 R5.1
N$5
  Top 0.152: Q1.5 115.25,18.54 115.51,18.29 117.67,18.29 117.79,18.41 R4.1
N$6
  Top 0.152: R54.1 109.16,89.7 C37.1 109.86,90.45 U4.P8 110.69,91.07 110.81,91.19 111.06,91.19 111.19,91.06 U4.P7
N$7
  Bottom 0.152: J9.12 141.7,97.03 142.43,97.03 142.7,97.3 SPEED.1
N$8
  Bottom 0.152: J6.SHLD1 J6.SHLD3 105.09,1.25 | 105.09,1.25 J6.SHLD4 J6.SHLD2 | SHLD2.2 105.09,1.25
N$9
  Top 0.61: U8.AC3 R18.1
N$10
  Top 0.813: MEAS.3 F1.2
  Bottom 0.152: MEAS.3 MEAS.1
N$11
  Top 0.152: LOG_BTN.2 32.7,5.17 R27.1
N$12  (via drill 0.3)
  Top 0.152: R26.1 132.91,75.27 126.81,81.37 126.81,96.77 128.21,98.17 v140.14,98.17
  Bottom 0.152: v140.14,98.17 140.4,98.42 SPEED.2
N$13
  Top 0.318: L3.1 arc-90 67.75,86.96 67.68,87.03 C12.1 65.94,87 L2.2
N$14  (via drill 0.3)
  Top 0.152: R_SCL.2 70.84,17.36 v70.8,17.4
  Bottom 0.152: I2C.3 74.84,16.41 73.85,17.4 v70.8,17.4
N$15  (via drill 0.3)
  Top 0.152: R_SDA.2 78.5,17.36 v78.42,17.44
  Bottom 0.152: v78.42,17.44 77.95,17.44 76.92,16.41 I2C.1
N$16  (via drill 0.3)
  Top 0.152: R37.2 24.7,12.23 v24.7,5.71
  Bottom 0.152: v24.7,5.71 23.43,5.71 23.06,5.35 LOG.2
N$17
  Bottom 0.152: D12.ANODE_3 18.73,3.17 21.02,3.17 22.02,4.18 LOG.1
N$18
  Bottom 0.152: WIFI.1 D11.ANODE_2
N$19
  Top 0.254: R40.2 R35.2 C27.1
N$20
  Top 0.254: C28.1 R42.2 R41.2
N$21  (via drill 0.3)
  Top 0.152: R25.1 129.6,77.94 126.3,81.24 126.3,97.41 127.06,98.17 v127.19,98.17
  Bottom 0.152: v127.19,98.17 127.44,98.42 LINK.2
N$22
  Bottom 0.152: BT.1 D11.ANODE_1
N$23
  Top 0.152: U7.2 138.09,68.94 138.87,69.72 C33.1
  Top 0.254: C23.1 C33.1
N$24
  Top 0.152: C34.1 R24.1 R11.1 131.38,68.58 132.67,67.29 U7.10
N$25
  Top 0.152: R29.1 139.64,61.98 141.16,63.5 141.16,64.52 139.89,65.79 U7.28
N$26  (via drill 0.3)
  Top 0.152: R36.2 11.87,12.19 10.73,11.05 v9.33,11.05
  Bottom 0.152: v9.33,11.05 9.33,9.54 BT.2
N$27
  Top 0.61: LOAD.1 R45.2
N$28
  Bottom 0.152: RESET_SW.2 116.52,6.06 RESET.2
N$29
  Bottom 0.152: BOOT.2 139.38,5.17 BOOT_SW.2
N$30
  Top 0.152: U7.16 133.82,64.29 133.54,64.01 133.54,63.33 135.19,61.68 R30.2
N$31
  Top 0.152: U7.15 133.81,64.79 133.16,64.14 133.16,62.99 133.54,62.61 R31.2
N$32  (via drill 0.3)
  Top 0.152: R28.2 10.22,12.32 9.84,11.94 8.95,11.94 8.32,11.3 v8.32,8.26
  Bottom 0.152: v8.32,8.26 8.32,7.35 8.69,6.99 WIFI.2
N$33
  Top 0.152: R33.2 108.9,9.53 108.27,8.89 107.76,8.89 106.84,7.97 J6.B5
N$34
  Top 0.152: J6.A5 103.84,8.02 R34.2
N$35
  Bottom 0.152: PVT.1 22.02,6.72 21.02,5.71 18.73,5.71 D12.ANODE_2
N$36
  Bottom 0.152: RTK.1 22.02,9.26 21.02,8.26 18.73,8.26 D12.ANODE_1
N$37  (via drill 0.3)
  Top 0.152: R39.2 20.51,12.19 21.65,11.05 v23.05,11.05
  Bottom 0.152: v23.05,11.05 23.05,9.54 RTK.2
N$38  (via drill 0.3)
  Top 0.152: R38.2 22.16,12.06 22.54,11.68 23.56,11.68 24.07,11.18 v24.07,8.26
  Bottom 0.152: v24.07,8.26 23.43,8.26 23.06,7.89 PVT.2
N$39
  Top 0.152: R32.2 136.84,61.85 135.59,63.1 U7.18
N$40
  Bottom 0.152: J2.14 9.07,97.04 LINK2.1
N$41
  Bottom 0.152: J2.12 19.74,96.98 SPEED2.1
N$42  (via drill 0.3)
  Top 0.152: R_SCL_IO.2 v106.36,85.98
  Bottom 0.152: v106.36,85.98 106.51,86.13 I2C_IO.3
N$43  (via drill 0.3)
  Top 0.152: R_SDA_IO.2 v106.36,84.33
  Bottom 0.152: v106.36,84.33 106.64,84.05 I2C_IO.1
N$44  (via drill 0.3)
  Top 0.152: R59.2 8.57,12.19 7.81,11.43 v7.81,5.71
  Bottom 0.152: PWR.2 8.31,4.45 7.81,4.94 v7.81,5.71
N$45
  Bottom 0.152: PWR.1 D11.ANODE_3
N$142  (via drill 0.3)
  Top 0.152: v33.21,83.57 R7.1
  Bottom 0.152: v33.21,83.57 33.21,84.54 32.7,85.05 32.7,85.6 32.93,85.83 32.93,89.55 31.32,91.16 27.65,91.16 24.7,94.11 24.7,97.54 23.81,98.42 SPEED2.2
N$143  (via drill 0.3)
  Top 0.152: v33.21,85.22 R6.1
  Bottom 0.152: v33.21,85.22 33.21,89.66 31.43,91.44 27.89,91.44 25.08,94.25 25.08,97.79 22.54,100.33 14.92,100.33 13.02,98.42 LINK2.2
N$144
  Top 0.152: C29.1 R9.2 R8.2
N$145
  Top 0.152: C30.1 R10.2 R12.2
N$146  (via drill 0.3)
  Top 0.152: C35.1 C36.1 37.82,84.24 v37.78,84.2 | v38.29,80.14 38.44,79.99 U9.2
  Bottom 0.152: v37.78,84.2 37.78,80.64 v38.29,80.14
N$147  (via drill 0.3)
  Top 0.152: v39.94,73.28 40.79,73.28 41.97,72.1 R13.1 R14.1 C40.1 | U9.10 40.34,74.91 v40.45,74.8
  Bottom 0.152: v40.45,74.8 39.94,74.3 v39.94,73.28
N$148
  Top 0.152: U9.28 41.84,81.91 42.23,82.3 42.86,82.3 44.01,83.44 R15.1
PW1+  (via drill 0.3)
  Top 1.905: PW+.3 9.84,72.9 | 9.84,72.9 9.84,70.36 9.91,70.29 U10.6 | U10.5 9.91,72.83 9.84,72.9
  Bottom 0.152: PW+.3 PW+.1
  other vias: 9.84,68.58 11.11,68.58 9.84,67.31 9.84,66.04 9.84,64.77 11.11,64.77 11.11,66.04 11.11,67.31 10.48,67.94 9.21,67.94 9.21,66.67 9.21,65.41 9.21,64.14 10.48,64.14 10.48,65.41 10.48,66.67
  pour Top (isolate 0.406): 8.95,71.12 11.49,71.12 11.49,63.75 8.95,63.75
  pour Bottom (isolate 0.406): 8.83,68.96 11.49,68.96 11.49,63.75 8.83,63.75
PW1-  (via drill 0.3)
  Top 0.152: v8.57,59.69 7.3,59.69
  Top 1.905: PW-.3 7.3,59.69 7.3,56.77 | 7.3,56.77 7.3,54.23 7.36,54.17 U10.8 | U10.7 7.36,56.71 7.3,56.77
  Bottom 0.152: PW-.3 PW-.1
  other vias: 8.57,62.23 9.84,62.23 11.11,62.23 9.84,60.96 8.57,60.96 8.57,58.42 9.84,58.42 11.11,58.42 11.11,59.69 9.84,59.69 11.11,60.96 10.48,61.59 9.21,61.59 10.48,60.33 9.21,60.33 9.21,59.05 10.48,59.05
  pour Top (isolate 0.406): 7.3,62.61 11.49,62.61 11.49,57.15 7.3,57.15
  pour Bottom (isolate 0.406): 8.19,62.61 11.49,62.61 11.49,58.04 8.19,58.04
PW+
  Bottom 0.152: PW+.4 PW+.2
  Bottom 1.905: J2.9 9.84,82.68 PW+.4
PW-
  Bottom 0.152: PW-.4 PW-.2
  Bottom 1.905: PW-.4 7.3,83.95 J2.10
RD+_ESP32  (via drill 0.3)
  Top 0.254: J9.3 140.02,81.92 139.28,81.17 D7.4 138.3,79.69 v138.11,79.5 | v137.86,75.82 R42.1 | U7.5 136.59,70.23 v136.72,70.36
  Bottom 0.254: v138.11,79.5 137.48,78.87 137.48,76.2 v137.86,75.82 137.86,71.5 v136.72,70.36
RD+_MOSAIC  (via drill 0.3)
  Top 0.152: R12.1 35.22,77.79 37.08,77.79 37.79,78.49 U9.5
  Top 0.254: v29.27,74.95 29.21,75.01 D1.1 | v33.08,76.96 R12.1
  Bottom 0.254: J2.3 18.1,81.41 24.55,74.95 v29.27,74.95 31.84,74.95 33.08,76.2 v33.08,76.96
RD-_ESP32  (via drill 0.3)
  Top 0.254: D7.6 138.18,77.79 v138.11,77.72 138.11,76.96 v139.51,75.56 R41.1 | U7.4 137.09,69.85 137.73,70.48 v139.51,70.48
  Bottom 0.254: J9.6 137.35,84.71 137.99,84.71 138.75,83.95 138.75,78.36 v138.11,77.72 | v139.51,70.48 v139.51,75.56
RD-_MOSAIC  (via drill 0.3)
  Top 0.152: U9.4 39.2,78.97
  Top 0.254: D1.3 31.11,74.61 v31.31,74.42 32.19,74.42 33.08,75.31 R10.1 | 39.2,78.97 v38.39,78.97
  Bottom 0.254: J2.6 15.43,84.71 16.07,84.71 16.83,83.95 16.83,82.04 24.45,74.42 v31.31,74.42 32.19,74.42 33.97,76.2 38.42,76.2 39.05,76.83 39.05,78.31 v38.39,78.97
RDY
  Top 0.152: U8.A12 RDY.1
REF
  Top 0.152: U8.AC17 U8.AC16 78.42,87.63 REF.1
SD_CLK  (via drill 0.3)
  Top 0.152: U8.AA1 93.79,81.28 v95.44,79.63
  Top 0.406: v44.53,13.98 44.52,13.98 J3.5 | v53.78,14.48 D32.1
  Bottom 0.152: v95.44,79.63 95.47,79.63 96.46,78.64 96.46,52.32 58.61,14.48 v53.78,14.48
  Bottom 0.406: v44.53,13.98 50.24,13.98 50.74,14.48 v53.78,14.48
SD_CMD  (via drill 0.3)
  Top 0.152: v95.95,80.39 93.79,82.55 U8.AB1 | D33.1 50.5,15.66 R46.1 v52.13,13.84
  Top 0.406: J3.3 46.72,14.15 47.05,14.48 50.1,14.48 50.48,14.86 D33.1
  Bottom 0.152: v95.95,80.39 95.95,79.54 96.74,78.76 96.74,52.09 58.48,13.84 v52.13,13.84
SD_DAT3
  Top 0.152: J3.2 47.82,13.72 48.07,13.97 50.86,13.97 51.5,13.34 54.04,13.34 55.44,14.73 R17.1
SD_DATA  (via drill 0.3)
  Top 0.152: 41.05,15.66 R47.1 | U8.Y1 v94.93,78.74 | D31.1 41.03,15.68
  Top 0.406: J3.7 42.32,13.62 42.1,13.84 39.94,13.84 39.31,14.48 D31.1 | 41.03,15.68 41.05,15.66 | R47.1 41.08,15.53 v41.08,14.48
  Bottom 0.152: v41.08,14.48 49.72,14.48 50.36,15.11 58.74,15.11 96.1,52.48 96.1,77.58 94.95,78.74 v94.93,78.74
SHIELD
  Bottom 0.152: J1.SHLD1 J1.SHLD3 127.95,1.25 | 127.95,1.25 J1.SHLD4 J1.SHLD2 | SHLD1.2 127.95,1.25
SPEED_ESP32  (via drill 0.3)
  Top 0.254: v133.67,71.5 133.67,72.05 R26.2 R57.2 | v140.14,67.31 140.12,67.29 U7.31
  Bottom 0.152: v133.67,71.5 137.86,67.31 v140.14,67.31
SPEED_MOSAIC  (via drill 0.3)
  Top 0.152: R7.2 36.89,83.57 37.91,82.55 40.29,82.55 v40.31,82.53 40.34,82.5 U9.31 | v46.8,84.2 46.76,84.24 R55.2
  Bottom 0.152: v40.31,82.53 41.21,83.44 46.04,83.44 v46.8,84.2
TD+_ESP32  (via drill 0.3)
  Top 0.254: R35.1 v142.81,75.56 142.81,76.67 143.83,77.69 143.83,79.12 143.26,79.69 D7.3 142.03,80.62 142.56,81.15 J9.1 | U7.7 135.59,68.94 135.45,69.09 135.45,70.99 136.1,71.65 142.66,71.65 v142.81,71.5
  Bottom 0.254: v142.81,71.5 v142.81,75.56
TD+_MOSAIC  (via drill 0.3)
  Top 0.254: v28.26,78.23 29.15,78.23 29.21,78.3 D1.6 | v33.08,78.61 R8.1 | v38.39,77.09 38.79,77.49 U9.7
  Bottom 0.254: J2.1 22.03,81.92 22.03,79.88 23.69,78.23 v28.26,78.23 32.7,78.23 v33.08,78.61 36.87,78.61 v38.39,77.09
TD-_ESP32  (via drill 0.3)
  Top 0.254: J9.2 141.29,81.53 140.91,81.15 140.91,77.85 141.03,77.72 141.96,77.72 D7.1 142.03,76.43 v141.16,75.56 R40.1 | U7.6 136.09,69.08 135.95,69.22 135.95,70.74 136.33,71.12 v141.16,71.12
  Bottom 0.254: v141.16,71.12 v141.16,75.56
TD-_MOSAIC  (via drill 0.3)
  Top 0.152: 38.44,77.99 v38.42,78.01
  Top 0.254: D1.4 32.05,78.84 v32.07,78.87 33.46,80.26 R9.1 | U9.6 38.44,77.99
  Bottom 0.254: J2.2 19.88,85.85 22.54,83.19 22.54,80.01 23.69,78.87 v32.07,78.87 32.58,79.38 37.05,79.38 v38.42,78.01
V_POE
  Top 0.61: LOAD.2 41.59,51.55
  Top 0.813: L1.2 38.19,51.68 C47.1 40.32,51.55 41.59,51.55 VPOE.1 D9.A
V_USB  (via drill 0.3, 0.5)
  Top 0.152: D10.5 127.95,13.72 128.21,13.97 129.22,13.97 129.73,13.46 129.73,9.31 v128.97,8.55
  Top 0.61: J1.VBUS2 130.4,7.53 v130.49,7.62 | J1.VBUS1 125.5,7.53 v125.41,7.62
  Top 0.813: VUSB.1 D5.A
  Route15 0.813: v125.41,7.62 126.34,8.55 v128.97,8.55 129.57,8.55 v130.49,7.62
  Route15 1.905: VUSB.1 40.7,43.18 38.16,40.64 33.97,40.64 31.56,38.23 31.56,20.07 42.74,8.89 51.75,8.89 65.72,22.86 91.12,22.86 102.55,11.43 121.6,11.43 v125.41,7.62
V_USB_2  (via drill 0.3, 0.5)
  Top 0.152: D8.5 v105.09,8.76
  Top 0.61: v107.63,7.62 107.54,7.53 J6.VBUS2 | J6.VBUS1 102.64,7.53 v102.55,7.62
  Top 0.813: VUSB2.1 D6.A
  Route15 0.813: v102.55,7.62 103.7,8.76 v105.09,8.76 106.49,8.76 v107.63,7.62
  Route15 1.905: v102.55,7.62 89.85,20.32 66.99,20.32 53.02,6.35 41.59,6.35 28.89,19.05 28.89,39.37 32.7,43.18 37.02,43.18 39.56,45.72 VUSB2.1
VANT
  Top 0.61: U8.P23 U8.R23 64.45,73.66 64.07,73.28 61.62,73.28 FB3.2
VCCA  (via drill 0.3)
  Top 0.254: v137.73,69.47 137.73,69.06 137.59,68.92 U7.3
  Top 0.406: J9.4 138.75,84.58 J9.5 137.48,78.74 | 137.48,78.74 D7.5 | C22.1 v134.56,75.82 135.32,76.58 136.72,76.58 137.48,77.34 137.48,78.74
  Top 0.813: FB2.2 144.59,62.1 VCCA.1 144.55,62.32 C38.1 C39.1
  Route15 0.406: VCCA.1 143.19,63.5 139.38,63.5 137.73,65.15 v137.73,69.47 137.73,70.61 134.56,73.79 v134.56,75.82
VCCIO  (via drill 0.3)
  Top 0.152: R23.1 99.72,91.53 v100.14,91.95
  Top 0.254: U17.8 100.53,91.56 v100.14,91.95 | U11.8 92.91,91.42 v92.93,91.44 | U15.8 49.39,90.38 v48.58,91.19 | U13.8 52.82,90.38 v52.01,91.19 | U14.8 45.07,90.38 44.89,90.55 v44.89,91.19 | U16.8 96.41,90.38 v95.76,89.72 | U18.8 103.36,90.38 v103.31,90.42
  Top 0.406: C59.1 v57.72,80.52
  Top 0.813: v39.83,91.19 v39.83,88.9 C45.1 C44.1 37.98,90.69 D29.1 37.98,93.42 38.88,94.32 J5.7 | R54.2 v107.51,90.93 | C43.1 v113.86,90.93 | VCCIO.2 120.33,89.15 119.79,89.7 C55.1 | C55.1 119.9,90.79 D30.1 119.9,95.61 J13.2 | C55.1 C52.1 121.64,91.86 121.73,91.95 | v121.22,91.95 121.73,91.95 | 121.73,91.95 v122.11,91.95
  Route15 0.254: v92.93,91.44 95.19,89.19 95.19,89.15
  Route15 0.813: 113.86,91.95 107.51,91.95 | 107.51,91.95 103.57,91.95 | 103.57,91.95 v100.14,91.95 97.98,91.95 v95.76,89.72 95.19,89.15 74.99,68.96 65.98,68.96 57.72,77.22 v57.72,80.52 57.72,89.41 55.94,91.19 v52.01,91.19 v48.58,91.19 v44.89,91.19 v39.83,91.19 v39.83,88.9 | v103.31,90.42 103.31,91.69 103.57,91.95 | v107.51,90.93 107.51,91.95 | v113.86,90.93 113.86,91.95 | v122.11,91.95 v121.22,91.95 113.86,91.95
  Bottom 0.152: I2C_IO.2 106.36,85.09 103.31,88.14 v103.31,90.42
VDDA  (via drill 0.3)
  Top 0.254: v37.78,79.5 39.21,79.5 U9.3
  Top 0.406: D1.5 v30.16,80.01 | C26.1 v30.16,80.01 | v30.16,80.01 18.86,80.01 J2.5 16.83,84.58 J2.4
  Top 0.61: C13.1 C24.1 47.05,70.32 | 47.05,70.32 FB1.2 | VDDA.1 47.05,66.42 47.05,70.32
  Route15 0.406: v30.16,80.01 37.27,80.01 v37.78,79.5 37.78,73.53 35.24,70.99 35.24,67.06 36.26,66.04 VDDA.1
VIN
  Top 0.813: L4.2 43.64,35.71 C85.1 44.25,38.34 D4.A VIN.1
VIN1+  (via drill 0.5)
  Top 1.905: v12.38,44.45 11.75,43.81 D14.A | v12.38,44.45 v12.38,43.18 11.74,43.18 D14.A | v12.38,44.45 11.74,44.45 D14.A
  Route15 1.905: VIN+.3 21.27,78.74 21.27,47.62 17.46,43.81 13.02,43.81 | 13.02,43.81 v12.38,44.45 v12.38,43.18 13.02,43.81
  Bottom 0.152: VIN+.3 VIN+.1
VIN1-
  Top 1.27: C86.- 9.7,39.23 9.84,39.37
  Top 1.905: 9.84,39.37 U12.2
  Route15 1.905: VIN-.4 31.43,85.09 23.81,77.47 23.81,46.48 16.7,39.37 U12.2
  Bottom 0.152: VIN-.4 VIN-.2
VIN2+
  Top 1.905: D14.C 6.55,43.56 6.55,35.3 7.42,34.43 C86.+ 9.09,34.29 U12.3
VIN+
  Top 1.905: VIN+.4 28.89,90.93 28.38,91.44 J5.10
  Bottom 0.152: VIN+.4 VIN+.2
VIN-
  Top 1.905: VIN-.3 31.43,90.93 31.88,91.38 J5.9
  Bottom 0.152: VIN-.3 VIN-.1

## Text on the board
Top: 1
Route2: 2
Route15: 3
Bottom: v10 | 4
Measures: V-Score To V-Score | Dimensions / In Inches
tDocu: Controlled Impedance: JLC7628 / Material: TG155 / 4-Layers / Thickness: 1.6mm / Outer Copper: 1oz / Inner Copper: 0.5oz / Finish: ENIG / Red Solder Resist / White Silkscreen / No clean process | Paul Clark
